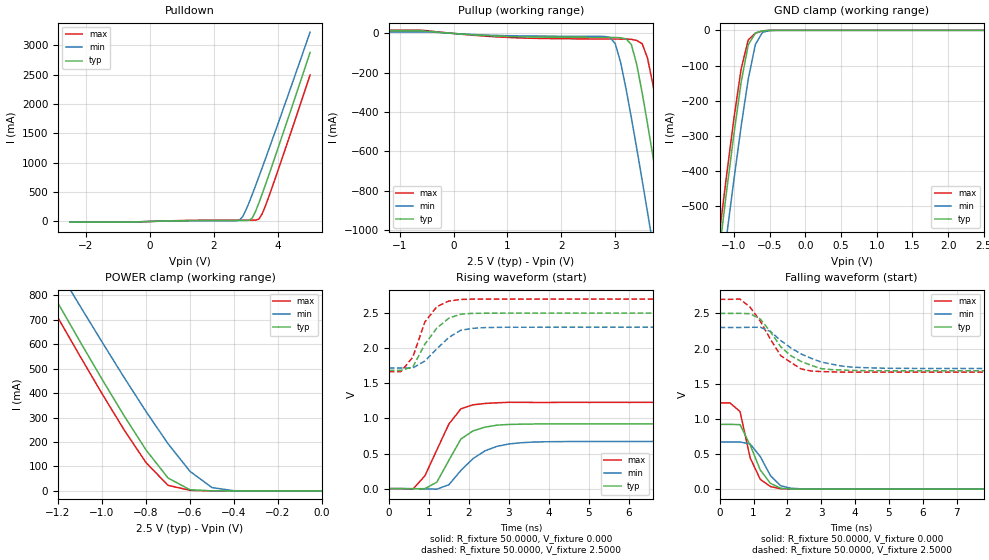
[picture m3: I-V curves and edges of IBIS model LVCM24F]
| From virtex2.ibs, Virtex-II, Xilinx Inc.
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|   Model LVCM24F
[Model]   LVCM24F
Model_type   I/O
Polarity   Non-Inverting
Enable   Active-Low
Vinh = 1.7V
Vinl = 0.7V
Vmeas =   1.2500V
Cref =  0pF
Rref =   1.0000M
Vref =  0.000V
C_comp   7.0000pF   6.0000pF   8.0000pF
[Temperature Range]   25.0000   100.0000   0.000
[Voltage Range]   2.5000V   2.3000V   2.7000V
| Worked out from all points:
|   slope of the pulldown table from 0 to 0.375 V, typ, clamps not added: 62.4 ohm
|   slope of the pullup table from 0 to 0.375 V, typ, clamps not added: 51.8 ohm
|   GND clamp passes 1 mA (typ) near -0.57 V on its own axis
|   POWER clamp passes 1 mA (typ) near -0.52 V on its own axis
|   rising waveform, R_fixture 50.0000, V_fixture 0.000: 20-80 % time 593ps typ, 782ps min, 635ps max; typ from 0 V to 0.922 V
|   rising waveform, R_fixture 50.0000, V_fixture 2.5000: 20-80 % time 601ps typ, 659ps min, 466ps max; typ from 1.68 V to 2.5 V
|   falling waveform, R_fixture 50.0000, V_fixture 0.000: 20-80 % time 552ps typ, 545ps min, 440ps max; typ from 0.922 V to 0 V
|   falling waveform, R_fixture 50.0000, V_fixture 2.5000: 20-80 % time 955ps typ, 1.22ns min, 845ps max; typ from 2.5 V to 1.68 V
[Pulldown]
| voltage   I(typ)   I(min)   I(max)
-2.5V     -10.76mA   -7.231mA   -12.39mA
-700mV    -10.76mA   -7.231mA   -12.39mA
2.8V      17.05mA    24.31mA    21.82mA
2.9V      17.1mA     87.6mA     21.85mA
3.1V      20.89mA    330.3mA    21.92mA
3.2V      63.97mA    469.9mA    22.14mA
3.3V      176mA      614.3mA    24.01mA
3.4V      314.9mA    761.4mA    40.63mA
3.5V      463.7mA    910.5mA    127.1mA
3.7V      773.9mA    1.212A     406.4mA
4V        1.252A     1.67A      874.2mA
5V        2.88A      3.228A     2.496A
[Pullup]
| voltage   I(typ)   I(min)   I(max)
-2.5V     13.18mA    7.45mA     16.56mA
2.9V      -20.4mA    -19.7mA    -28.22mA
3V        -20.58mA   -51.18mA   -28.34mA
3.1V      -21.73mA   -146.2mA   -28.45mA
3.3V      -56.22mA   -428.7mA   -29.9mA
3.4V      -157.9mA   -585.2mA   -35.79mA
3.6V      -459.5mA   -909.3mA   -125.5mA
3.7V      -624mA     -1.074A    -260.7mA
3.8V      -792.1mA   -1.241A    -416.5mA
4V        -1.134A    -1.577A    -748.3mA
4.2V      -1.481A    -1.916A    -1.09A
5V        -2.888A    -3.284A    -2.493A
[GND_clamp]
| voltage   I(typ)   I(min)   I(max)
-2.5V     -2.881A    -2.936A    -2.838A
-1.2V     -617mA     -740.6mA   -570.6mA
-1.1V     -452.1mA   -579.7mA   -406.1mA
-1V       -293.4mA   -423mA     -249mA
-900mV    -148mA     -273.4mA   -110.1mA
-800mV    -41mA      -138.5mA   -27.22mA
-700mV    -7.569mA   -40.19mA   -8.128mA
-600mV    -1.403mA   -5.589mA   -1.597mA
-500mV    -127.6uA   -662.5uA   -122uA
2.5V      397.5nA    2.548uA    351.3nA
[POWER_clamp]
| voltage   I(typ)   I(min)   I(max)
-2.5V     2.874A     2.908A     2.816A
-1.3V     925.8mA    1.055A     866.1mA
-1.2V     767.5mA    905.5mA    707.7mA
-1.1V     610.9mA    756.3mA    551.2mA
-1V       456.9mA    609.1mA    397.6mA
-900mV    307.7mA    464.5mA    250.2mA
-800mV    167.5mA    324.6mA    115.6mA
-700mV    52.75mA    192.9mA    22.81mA
-600mV    4.571mA    79.88mA    2.444mA
-500mV    271.3uA    13.45mA    251.8uA
-400mV    16.93uA    820.9uA    15.04uA
0V        397.5nA    368nA      428.7nA
[Ramp]
| variable   typ   min   max
dV/dt_r   0.5529/0.6437n   0.4028/0.7969n   0.7368/0.5442n
dV/dt_f   0.4896/0.9932n   0.3498/1.2320n   0.6210/0.8742n
R_load = 50.0000
[Rising Waveform]
R_fixture = 50.0000
V_fixture = 0.000
| time   V(typ)   V(min)   V(max)
0s        14.2uV     15.29uV    14.22uV
600ps     -2.697mV   -323.5uV   -7.758mV
900ps     -1.073mV   -4.203mV   181.1mV
1.2ns     91.78mV    -8.072mV   551.7mV
1.5ns     403.1mV    54.82mV    919.1mV
1.8ns     705.7mV    258mV      1.136V
2.1ns     821mV      425.8mV    1.193V
2.7ns     903.7mV    601.7mV    1.222V
3.6ns     920.2mV    662.6mV    1.228V
15ns      921.5mV    671.4mV    1.228V
[Rising Waveform]
R_fixture = 50.0000
V_fixture = 2.5000
V_fixture_min = 2.3000
V_fixture_max = 2.7000
| time   V(typ)   V(min)   V(max)
0s        1.684V     1.717V     1.665V
300ps     1.684V     1.717V     1.665V
600ps     1.734V     1.72V      1.874V
900ps     2.058V     1.817V     2.375V
1.2ns     2.287V     1.992V     2.592V
1.5ns     2.428V     2.154V     2.672V
1.8ns     2.486V     2.256V     2.695V
2.1ns     2.497V     2.284V     2.699V
3ns       2.5V       2.299V     2.699V
15ns      2.5V       2.3V       2.7V
[Falling Waveform]
R_fixture = 50.0000
V_fixture = 0.000
| time   V(typ)   V(min)   V(max)
0s        921.5mV    671.5mV    1.228V
300ps     921.5mV    671.5mV    1.228V
600ps     917.9mV    671.5mV    1.105V
900ps     627.4mV    642.7mV    444.9mV
1.2ns     271.7mV    462.8mV    138.8mV
1.5ns     82.04mV    191.8mV    36.99mV
1.8ns     14.31mV    48.85mV    5.789mV
2.1ns     2.491mV    13.92mV    321.7uV
3ns       21.79uV    455.8uV    74.22uV
15ns      13.3uV     5.914uV    10.96uV
[Falling Waveform]
R_fixture = 50.0000
V_fixture = 2.5000
V_fixture_min = 2.3000
V_fixture_max = 2.7000
| time   V(typ)   V(min)   V(max)
0s        2.5V       2.3V       2.7V
600ps     2.501V     2.3V       2.704V
900ps     2.495V     2.303V     2.588V
1.2ns     2.42V      2.303V     2.388V
1.8ns     2.027V     2.115V     1.9V
2.4ns     1.818V     1.925V     1.711V
2.7ns     1.762V     1.861V     1.681V
3.6ns     1.694V     1.752V     1.665V
4.8ns     1.685V     1.721V     1.665V
15ns      1.684V     1.717V     1.665V
